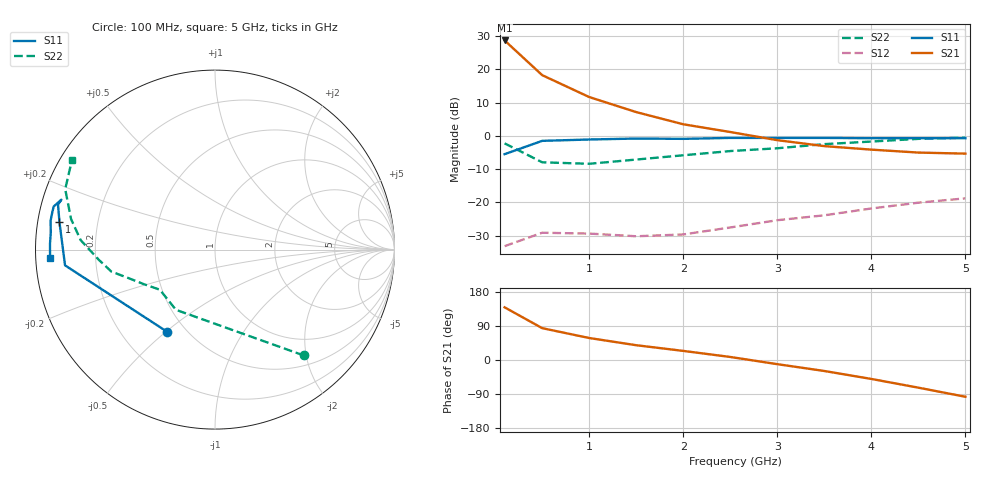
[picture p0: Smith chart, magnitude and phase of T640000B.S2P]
!AT-64000
!S-PARAMETERS at Vce=16V  Ic=110mA.  LAST UPDATED 07-13-94
# ghz s ma r 50
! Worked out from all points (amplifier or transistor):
!   11 points, 100 MHz to 5 GHz, reference 50 ohm
!   highest |S21| = 28.6 dB at 100 MHz (marker M1)
!   |S21| within 3 dB of that: start of sweep to 215 MHz
!   unconditionally stable (mu >= 1): 1.992 GHz to 2.008 GHz; 4.822 GHz to end of sweep
!   at 500 MHz: K = 0.29, MSG = 23.7 dB, |S12| = -29.1 dB
!   at 2.5 GHz: K = 0.50, MSG = 14.3 dB, |S12| = -27.5 dB
!   at 5 GHz: K = 1.02, MAG = 5.8 dB, |S12| = -18.8 dB
!   S11 on the Smith chart (normalised r, x): 100 MHz: 0.40, -0.51; 1 GHz: 0.06, +0.09; 5 GHz: 0.04, -0.03
0.1  0.53 -120.0  27.05 139.0  0.022 43.0  0.77 -50.0
0.5  0.84 -174.0  8.14 84.0  0.035 12.0  0.4 -123.0
1  0.88 170.0  3.82 58.0  0.034 -4.0  0.38 -144.0
1.5  0.91 164.0  2.27 39.0  0.031 -16.0  0.44 -154.0
2  0.9 162.0  1.49 24.0  0.033 -38.0  0.51 -162.0
2.5  0.93 165.0  1.14 8.0  0.042 -47.0  0.59 -168.0
3  0.93 167.0  0.86 -11.0  0.054 -61.0  0.65 -175.0
3.5  0.93 170.0  0.7 -29.0  0.064 -75.0  0.75 176.0
4  0.92 174.0  0.62 -50.0  0.081 -83.0  0.82 168.0
4.5  0.92 178.0  0.56 -73.0  0.099 -93.0  0.9 158.0
5  0.92 -177.0  0.54 -97.0  0.115 -101.0  0.94 148.0
